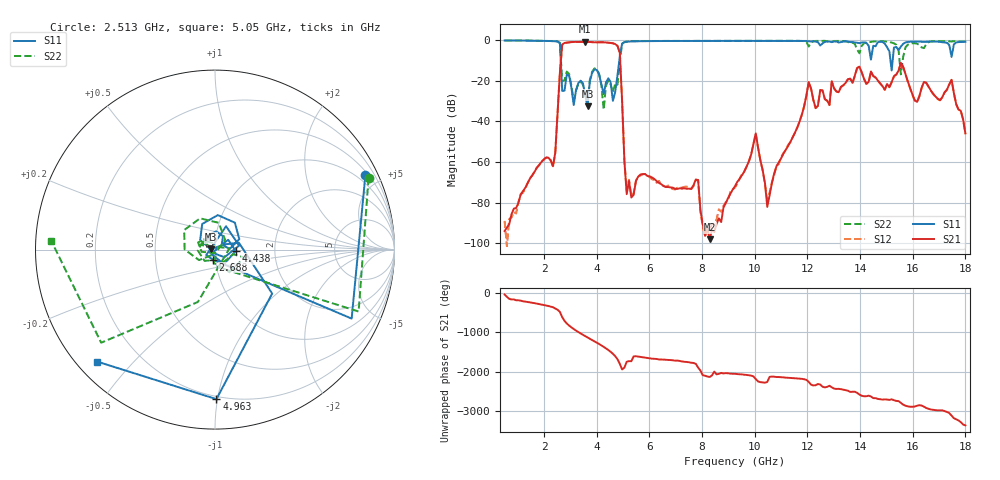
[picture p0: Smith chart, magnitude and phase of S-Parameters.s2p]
!Agilent Technologies,N5230A,MY45001468,A.07.50.67
!Agilent N5230A: A.07.50.67
!Date: Thursday, June 27, 2024 10:30:33
!Correction: S11(Full 2 Port(1,2))
!S21(Full 2 Port(1,2))
!S12(Full 2 Port(1,2))
!S22(Full 2 Port(1,2))
!S2P File: Measurements: S11, S21, S12, S22:
# Hz S  dB  R 50
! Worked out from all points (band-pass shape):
!   201 points, 500 MHz to 18 GHz, reference 50 ohm
!   highest |S21| = -0.69 dB at 3.562 GHz (marker M1); lowest = -98.1 dB at 8.287 GHz (marker M2)
!   |S21| within 3 dB of the highest: 2.677 GHz to 4.813 GHz (2.136 GHz wide, 57 % of centre)
!   lowest |S11| = -32.5 dB at 3.65 GHz (marker M3), VSWR 1.05, Z = 47.7 + j0.189 ohm
!   |S11| at or under -10 dB: 2.632 GHz to 4.855 GHz (2.223 GHz wide, 59.4 % of centre); 15.16 GHz to 15.24 GHz (81.85 MHz wide, 0.539 % of centre)
!   |S22| runs from -34.1 to 0.0 dB; largest |S21 - S12| = 0.0038
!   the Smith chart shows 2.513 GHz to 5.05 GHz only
!   S11 on the Smith chart (normalised r, x): 2.513 GHz: 0.64, +4.18; 2.688 GHz: 0.97, -0.11; 4.438 GHz: 1.26, -0.02; 4.963 GHz: 0.18, -0.99; 5.05 GHz: 0.06, -0.40
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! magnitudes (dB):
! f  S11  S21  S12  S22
! 500 MHz  0.0  -94.1  -89.1  0.0
! 2.337 GHz  -0.4  -62.1  -62.2  -0.3
! 2.513 GHz  -0.6  -36.0  -36.0  -0.5
! 2.688 GHz  -24.9  -2.1  -2.1  -20.2
! 3.475 GHz  -21.2  -0.7  -0.7  -21.8
! 3.562 GHz  -27.2  -0.7  -0.7  -28.6
! 3.65 GHz  -32.5  -0.7  -0.7  -30.2
! 4.438 GHz  -18.7  -1.1  -1.1  -19.8
! 4.875 GHz  -7.9  -6.2  -6.2  -10.3
! 4.963 GHz  -1.6  -30.0  -30.0  -1.7
! 5.05 GHz  -0.9  -59.6  -59.6  -0.8
! 6.362 GHz  -0.3  -70.3  -69.3  -0.3
! 8.287 GHz  -0.2  -98.1  -93.3  -0.2
! 9.25 GHz  -0.2  -71.9  -72.6  -0.2
! 10.04 GHz  -0.3  -45.8  -45.9  -0.2
! 10.47 GHz  -0.2  -82.2  -78.7  -0.2
! 12.22 GHz  -0.5  -29.3  -29.4  -0.4
! 15.11 GHz  -5.4  -23.0  -23.1  -0.7
! 15.55 GHz  -3.0  -11.1  -11.2  -16.7
! 16.16 GHz  -0.6  -30.3  -30.5  -1.6
! 17.48 GHz  -8.1  -19.4  -19.6  -0.5
! 18 GHz  -0.7  -45.9  -46.1  -0.5
